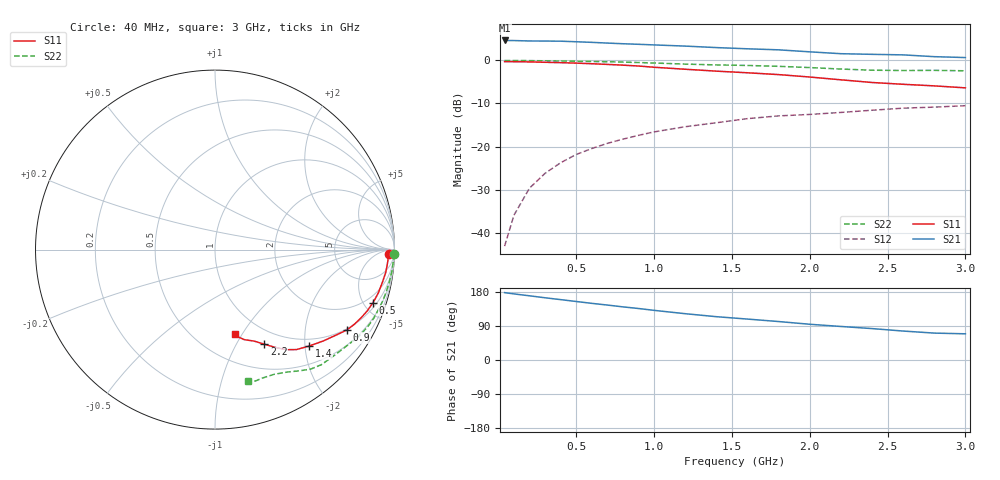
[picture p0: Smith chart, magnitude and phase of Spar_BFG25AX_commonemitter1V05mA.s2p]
! Filename:  BFG25AXC.S2P  Version:  2.0
! NXP part #: BFG25A/X  Date: May 1990
! Bias condition: Vce=1V, Ic=0.5mA
#  MHz  S  MA  R  50
! Freq  S11  S21  S12  S22  !GUM [dB]
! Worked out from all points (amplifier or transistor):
!   21 points, 40 MHz to 3 GHz, reference 50 ohm
!   highest |S21| = 4.6 dB at 40 MHz (marker M1)
!   |S21| within 3 dB of that: start of sweep to 2.167 GHz
!   unconditionally stable (mu >= 1): nowhere
!   at 300 MHz: K = 0.10, MSG = 15.3 dB, |S12| = -26.2 dB
!   at 1 GHz: K = 0.29, MSG = 10.1 dB, |S12| = -16.6 dB
!   at 3 GHz: K = 0.73, MSG = 5.6 dB, |S12| = -10.5 dB
!   lowest NFmin = 1.40 dB at 500 MHz
!   S11 on the Smith chart (normalised r, x): 40 MHz: 37, -29; 500 MHz: 1.36, -5.83; 900 MHz: 0.96, -3.30; 1.4 GHz: 0.85, -2.08; 2.2 GHz: 0.80, -1.31; 3 GHz: 0.76, -0.92
40  0.967 -1.5  1.702 177.8  0.007 85.6  0.997 -1.4
100  0.965 -3.9  1.697 174.4  0.016 86.9  0.996 -3.5
200  0.96 -7.5  1.679 169.4  0.033 84.2  0.993 -6.9
300  0.95 -11.2  1.675 164.2  0.049 81.7  0.988 -10.4
400  0.941 -15.0  1.669 159.3  0.065 79.0  0.983 -13.7
500  0.929 -18.5  1.644 154.4  0.081 76.5  0.977 -17.1
600  0.914 -22.0  1.618 149.5  0.095 74.5  0.97 -20.2
700  0.898 -25.1  1.587 145.0  0.109 72.4  0.964 -23.3
800  0.88 -28.3  1.559 140.2  0.122 70.3  0.955 -26.2
900  0.86 -31.4  1.536 135.9  0.135 68.4  0.944 -29.0
1000  0.832 -34.5  1.511 131.0  0.148 66.1  0.932 -31.8
1200  0.789 -40.2  1.464 122.2  0.17 61.4  0.905 -37.1
1400  0.75 -45.8  1.407 114.3  0.189 58.3  0.886 -42.4
1600  0.718 -50.9  1.362 108.0  0.211 55.8  0.873 -47.3
1800  0.684 -54.6  1.325 101.5  0.227 52.5  0.853 -51.3
2000  0.641 -58.3  1.256 94.3  0.236 49.7  0.825 -54.9
2200  0.595 -62.4  1.195 88.5  0.249 47.1  0.793 -59.3
2400  0.554 -66.9  1.175 82.9  0.264 43.7  0.769 -64.6
2600  0.528 -71.9  1.158 76.4  0.279 40.2  0.763 -69.5
2800  0.506 -74.8  1.104 71.0  0.287 39.0  0.766 -73.1
3000  0.48 -76.9  1.078 69.1  0.298 38.6  0.757 -75.9
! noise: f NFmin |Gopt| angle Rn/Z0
500  1.4  0.89  5  2.8
1000  1.6  0.8  14  3
2000  1.8  0.75  39  2.1
